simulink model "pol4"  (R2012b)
settings: Solver=ode45  StartTime=0.0  StopTime=10.0  RelTol=1e-3
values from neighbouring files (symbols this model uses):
  A = [0 1 0 0 0 0    [beobachter_1.m]    (also in beobachter_2.m; beobachter_22.m; kalman_1.m = my_sys.a; kalman_10.m = my_sys.a)
  B = [0 1 0 0 0 0]'    [beobachter_1.m]    (also in beobachter_2.m; beobachter_22.m; kalman_1.m = my_sys.b; kalman_10.m = my_sys.b)
  C = [0 0 0 0 1 0]    [beobachter_1.m]    (also in beobachter_2.m; beobachter_22.m; kalman_1.m = my_sys.c; kalman_10.m = my_sys.c)
  D = 0    [aktiv_tilger_1.m]    (also in aktiv_tilger_12.m; aktiv_tilger_3.m = 2000; aktiv_tilger_31.m; beobachter_1.m)
  K = Kn(1:n)    [beobachter_2.m]    (also in beobachter_22.m; LQG_1.m = lqry(sys,10,1); LQR_1.m = Kn(1:6),      ki = -Kn(7),; pol_4.m)
  ki = -Kn(n+1)    [beobachter_2.m]    (also in beobachter_22.m; kalman_12.m = -Kn(3); kalman_13.m = -Kn(4); kalman_d1.m = -Kn(4))

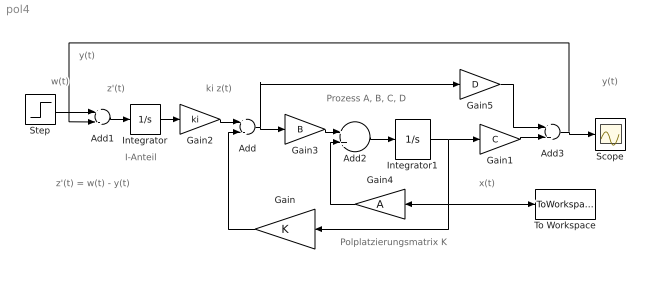
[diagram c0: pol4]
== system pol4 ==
  note: z'(t) = w(t) - y(t)
  note: y(t)
  note: w(t)
  note: ki z(t)
  note: z'(t)
  note: y(t)
  note: x(t)
  note: I-Anteil
  note: Polplatzierungsmatrix K
  note: Prozess A, B, C, D
  Add : Sum  Inputs=+-
  Add1 : Sum  Inputs=+-
  Add2 : Sum
  Add3 : Sum
  Gain : Gain  Gain=K  Multiplication=Matrix(K*u)
  Gain1 : Gain  Gain=C  Multiplication=Matrix(K*u)
  Gain2 : Gain  Gain=ki
  Gain3 : Gain  Gain=B  Multiplication=Matrix(K*u)
  Gain4 : Gain  Gain=A  Multiplication=Matrix(K*u)
  Gain5 : Gain  Gain=D  Multiplication=Matrix(K*u)
  Integrator : Integrator
  Integrator1 : Integrator
  Scope : Scope
  Step : Step  SampleTime=0
  To Workspace : ToWorkspace  VariableName=x  SampleTime=-1  SaveFormat=Structure With Time
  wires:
  Integrator1/1 -> Gain1/1, To Workspace/1, Gain/1, Gain4/1
  Gain/1 -> Add/2
  Add1/1 -> Integrator/1
  Step/1 -> Add1/1
  Gain1/1 -> Add3/2
  Integrator/1 -> Gain2/1
  Gain2/1 -> Add/1
  Add2/1 -> Integrator1/1
  Gain3/1 -> Add2/1
  Gain4/1 -> Add2/2
  Add3/1 -> Add1/2, Scope/1
  Add/1 -> Gain5/1, Gain3/1
  Gain5/1 -> Add3/1
